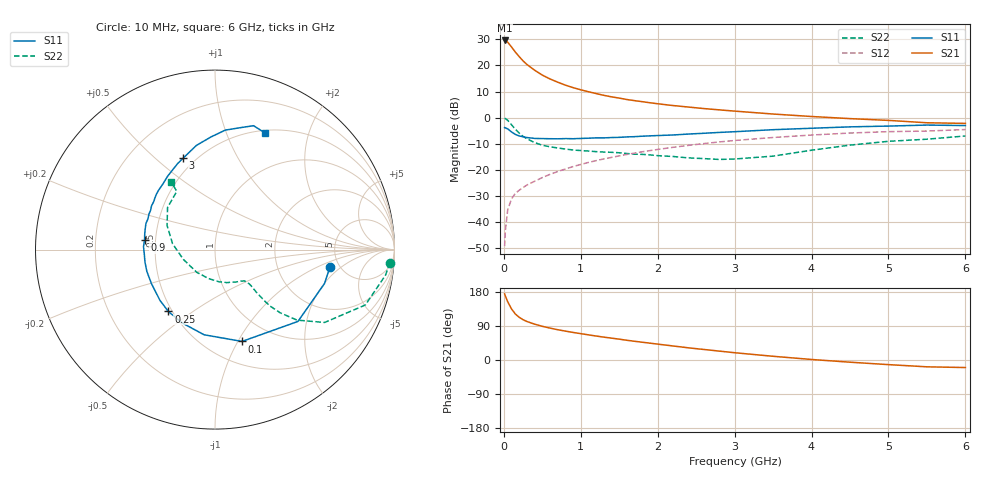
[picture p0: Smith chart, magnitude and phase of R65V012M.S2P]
! SIEMENS Small Signal Semiconductors
! BFR193
! Si NPN RF Bipolar Junction Transistor in SOT23
! VCE = 5 V  IC = 12 mA
! Common Emitter S-Parameters:  May  1996
# GHz  S  MA  R  50
!  f  S11  S21  S12  S22
! GHz  MAG  ANG  MAG  ANG  MAG  ANG  MAG  ANG
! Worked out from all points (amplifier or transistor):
!   36 points, 10 MHz to 6 GHz, reference 50 ohm
!   highest |S21| = 29.5 dB at 10 MHz (marker M1)
!   |S21| within 3 dB of that: start of sweep to 112.8 MHz
!   unconditionally stable (mu >= 1): 700.8 MHz to 1.979 GHz
!   at 250 MHz: K = 0.69, MSG = 24.2 dB, |S12| = -26.7 dB
!   at 1.4 GHz: K = 1.04, MAG = 10.4 dB, |S12| = -15.2 dB
!   at 6 GHz: K = 0.94, MSG = 1.2 dB, |S12| = -4.5 dB
!   S11 on the Smith chart (normalised r, x): 10 MHz: 4.17, -1.41; 100 MHz: 0.73, -1.04; 250 MHz: 0.48, -0.40; 900 MHz: 0.43, +0.06; 3 GHz: 0.43, +0.62; 6 GHz: 0.53, +1.37
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0.01  0.6473 -8.7  29.96 174.4  0.0035 86.7  0.9772 -4.3
0.02  0.6389 -17.2  29.51 168.8  0.007 81.4  0.9609 -8.5
0.05  0.6113 -40.9  27.77 153.8  0.0172 73.7  0.8929 -20.2
0.1  0.5333 -73.6  22.47 134.7  0.0281 63.6  0.7334 -33.6
0.15  0.4784 -97.3  17.92 121.3  0.0357 58.8  0.6024 -40.7
0.2  0.4477 -114.1  14.68 112.6  0.0411 57.8  0.5058 -44.1
0.25  0.4317 -127.0  12.18 106.3  0.0462 57.4  0.4393 -45.7
0.3  0.4174 -137.2  10.41 101.6  0.0517 58.4  0.3956 -46.0
0.4  0.4017 -151.8  8.089 94.6  0.0609 60.5  0.3344 -45.9
0.5  0.3986 -162.2  6.519 88.9  0.0717 62.3  0.2978 -45.3
0.6  0.3963 -169.9  5.503 84.2  0.0826 63.5  0.2781 -45.0
0.7  0.3947 -176.6  4.776 79.9  0.0934 64.0  0.2638 -45.2
0.9  0.3963 172.1  3.757 72.7  0.1164 64.5  0.2411 -46.5
1.1  0.4056 163.4  3.132 66.3  0.1395 64.0  0.2303 -49.7
1.3  0.4108 155.5  2.676 60.3  0.1628 62.9  0.2203 -53.3
1.6  0.4295 145.4  2.224 52.0  0.1984 60.4  0.2068 -61.2
2.2  0.4673 128.3  1.707 37.0  0.2716 54.1  0.1813 -82.4
3  0.5395 109.2  1.336 19.2  0.3669 43.2  0.1623 -128.8
3.5  0.5898 100.1  1.175 9.8  0.4183 35.7  0.1842 -162.6
4.5  0.6681 85.1  0.96 -5.8  0.5089 21.1  0.2991 153.2
5.5  0.723 72.7  0.8 -18.0  0.5555 6.0  0.388 123.3
6  0.7075 67.0  0.778 -19.9  0.5934 1.5  0.4474 122.9
